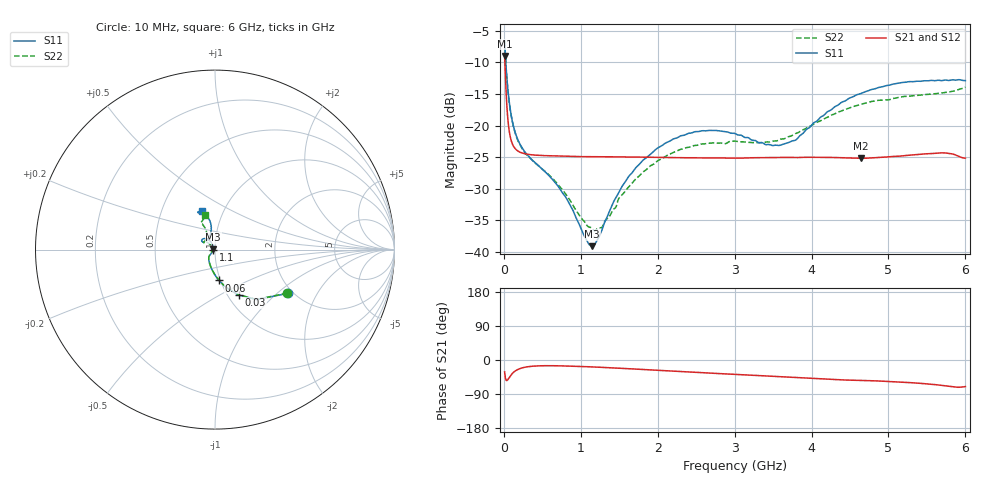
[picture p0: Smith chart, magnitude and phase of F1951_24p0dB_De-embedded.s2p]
! Integrated Device Technology
! Corporate Headquarters
! 6024 Silver Creek Valley Road
! San Jose, CA 95138  USA
! Phone:  1-408-284-8200
! Toll Free:  1-800-223-1366
! Webpage:  http://www.idt.com/
! Timing and RF Division
! 515 Groton Road, Suite 102
! Westford, MA 01886-6024
! Device:  F1951
! Description: 6-bit 0.5 dB Digital Step Attenuator
! Frequency:  100.0 -  4000.00 MHz
! Package:  4x4 mm Thin QFN Plastic Package: 24 pin
! Ports:  2 RF, 6 DC
!  Pin  1  = NC
!  Pin  2  = RF1  =  Port 1
!  Pin  3  = GND
!  Pin  4  = NC
!  Pin  5  = Serial Data Out (SDO)
!  Pin  6  = NC
!  Pin  7  = Reset Bar ( RSTb)
!  Pin  8  = Clock (CLK)
!  Pin  9  = Chip Select Bar (CSb)
!  Pin 10  = NC
!  Pin 11  = Serial Data In (SDI)
!  Pin 12  = NC
!  Pin 13  = NC
!  Pin 14  = VDD
!  Pin 15  = NC
!  Pin 16  = GND
!  Pin 17  = RF2  =  Port 2
!  Pin 18  = NC
!  Pin 19  = GND
!  Pin 20  = GND
!  Pin 21  = GND
!  Pin 22  = GND
!  Pin 23  = GND
!  Pin 24  = GND
! State:  48
! Atten State:  24.0 dB
! Voltage:  +3.30 Volts
! Current:  0.475 mA
! Data:  The device was measured on a F195X evaluation board which has
!  individual transmission lines to the RF pins.  Data was collected
!  de-embedded using a Automatic Fixture Removal [AFR] (Keysight Technologies).
!  The reference plane is the edge of the package pin.
! Misc:  Lot Code  1225BCA
!  Action Tracker AT0399
! Date Measured:  2018-09-13
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# GHz S dB R 50
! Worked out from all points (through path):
!   600 points, 10 MHz to 6 GHz, reference 50 ohm
!   highest |S21| = -8.98 dB at 10 MHz (marker M1); lowest = -25.2 dB at 4.64 GHz (marker M2)
!   group delay of S21, straight-line fit = 25.2 ps
!   lowest |S11| = -39.1 dB at 1.15 GHz (marker M3), VSWR 1.02, Z = 48.9 + j0.2 ohm
!   |S11| at or under -10 dB: 25.79 MHz to end of sweep
!   |S22| runs from -36.7 to -6.6 dB; largest |S21 - S12| = 0.0002
!   S11 on the Smith chart (normalised r, x): 10 MHz: 1.88, -1.18; 30 MHz: 1.13, -0.62; 60 MHz: 0.99, -0.35; 1.1 GHz: 0.98, -0.00; 6 GHz: 0.80, +0.36
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0.01  -6.51 -31.1  -8.98 -31.5  -8.98 -31.5  -6.56 -31.1
0.03  -10.86 -62.2  -14.84 -53.7  -14.84 -53.8  -10.91 -62.2
0.06  -15.21 -82.4  -19.95 -49.5  -19.95 -49.5  -15.29 -82.5
0.09  -17.98 -94.2  -22.13 -40.4  -22.13 -40.4  -18.04 -94.4
0.12  -19.87 -102.8  -23.16 -33.5  -23.16 -33.5  -19.91 -102.8
0.23  -23.38 -120.5  -24.33 -21.3  -24.32 -21.3  -23.50 -120.6
0.71  -29.69 -133.6  -24.83 -15.3  -24.83 -15.4  -29.45 -137.0
1.01  -36.57 -151.6  -24.93 -17.3  -24.93 -17.3  -34.75 -150.5
1.1  -38.70 -173.3  -24.94 -17.8  -24.94 -17.8  -36.06 -162.2
1.15  -39.13 169.3  -24.94 -18.3  -24.94 -18.3  -36.36 -171.5
1.27  -36.73 134.5  -24.95 -19.4  -24.95 -19.3  -36.18 164.7
1.6  -28.50 116.2  -24.99 -22.7  -24.99 -22.7  -30.06 134.7
2.01  -23.49 124.3  -25.05 -27.3  -25.05 -27.3  -25.51 135.4
2.49  -20.97 137.4  -25.12 -32.5  -25.12 -32.5  -23.15 142.8
3.01  -21.30 147.8  -25.17 -38.0  -25.17 -37.9  -22.47 146.3
3.58  -23.16 127.3  -25.05 -43.9  -25.05 -43.9  -22.26 129.3
3.79  -22.32 111.4  -25.08 -46.2  -25.08 -46.2  -21.29 122.3
4.01  -19.81 102.4  -25.03 -48.5  -25.03 -48.5  -19.92 116.9
4.64  -14.93 102.3  -25.19 -54.2  -25.19 -54.1  -16.65 115.7
5.01  -13.60 109.0  -24.95 -56.6  -24.95 -56.5  -15.91 117.5
5.71  -12.85 114.0  -24.33 -67.5  -24.33 -67.5  -14.81 110.6
6  -12.87 107.9  -25.16 -70.1  -25.16 -70.1  -13.92 106.7
